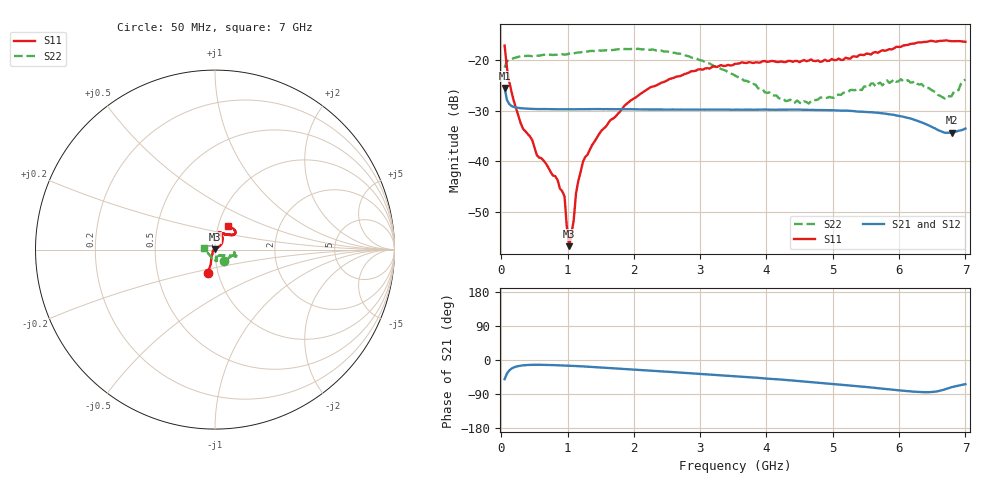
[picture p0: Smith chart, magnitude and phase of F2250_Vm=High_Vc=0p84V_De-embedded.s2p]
! Integrated Device Technology
! Corporate Headquarters
! 6024 Silver Creek Valley Road
! San Jose, CA 95138  USA
! Phone:  1-408-284-8200
! Toll Free:  1-800-223-1366
! Webpage:  http://www.idt.com/
! Timing and RF Division
! 515 Groton Road, Suite 102
! Westford, MA 01886-6024
! Device:  F2250
! Description: Voltage Variable RF Attenuator
! Frequency:  50.0 -  6000.00 MHz
! Package:  3x3 mm Thin QFN Plastic Package: 16 pin
! Ports:  2 RF, 3 DC
!  Pin  1  = GND
!  Pin  2  = NC
!  Pin  3  = RF1  = Port 1
!  Pin  4  = NC
!  Pin  5  = GND
!  Pin  6  = GND
!  Pin  7  = GND
!  Pin  8  = GND
!  Pin  9  = NC
!  Pin 10  = RF2  = Port 2
!  Pin 11  = NC
!  Pin 12  = GND
!  Pin 13  = GND
!  Pin 14  = VCNTRL
!  Pin 15  = VDD
!  Pin 16  = VMODE
! Vcntrl:  0.840 Volts
! Vmode:  +3.300 Volts
! Vdd:  +3.30  Volts
! Current:  1.308 mA
! Data:  The device was measured on a the F2250 evaluation board which has
!  individual transmission lines to the RF pins.  Data was collected
!  using a calibrated network analyzer.  The evaluation board was
!  de-embedded using a TRL calibration technique.
!  The reference plane is the edge of the package pin.
! Misc:  SN 10
!  Action Tracker AT0258
! Date Measured:  2014-11-26
! Date:  2015-10-15  MJV
! Note:
!  Integrated Device Technology supplies this data as a sample of measured
!  data at the package pin for this product.  Your particular data for this
!  product may vary.
!  Data was taken at 25 degrees C.
!  Integrated Device Technology reserves the right to change this data at anytime.
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# GHz S dB R 50
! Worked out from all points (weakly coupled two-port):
!   201 points, 50 MHz to 7 GHz, reference 50 ohm
!   highest |S21| = -25.53 dB at 50 MHz (marker M1); lowest = -34.4 dB at 6.792 GHz (marker M2)
!   lowest |S11| = -56.7 dB at 1.023 GHz (marker M3), VSWR 1.00, Z = 49.9 + j0.128 ohm
!   |S11| at or under -10 dB: start of sweep to end of sweep
!   |S22| runs from -28.6 to -17.8 dB; largest |S21 - S12| = 0.00014
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0.05  -17.15 -107.5  -25.53 -50.6  -25.52 -50.6  -21.52 -51.9
0.1195  -24.23 -110.3  -28.70 -27.7  -28.71 -27.7  -19.98 -15.0
0.29325  -32.52 -123.7  -29.53 -14.9  -29.50 -14.9  -19.22 -9.3
0.5365  -38.78 -149.6  -29.68 -12.7  -29.68 -12.7  -19.16 -9.0
0.8145  -42.95 171.8  -29.73 -13.6  -29.72 -13.6  -19.00 -12.1
0.9535  -46.90 174.9  -29.74 -14.5  -29.76 -14.5  -18.96 -13.8
0.98825  -52.90 169.1  -29.75 -14.8  -29.74 -14.8  -18.88 -14.2
1.023  -56.74 117.8  -29.74 -15.1  -29.72 -15.1  -18.76 -14.2
1.0925  -51.61 52.9  -29.73 -15.6  -29.73 -15.6  -18.70 -14.7
1.12725  -46.27 41.7  -29.73 -15.9  -29.72 -15.9  -18.59 -15.2
1.2315  -40.09 32.1  -29.72 -16.9  -29.72 -16.9  -18.39 -16.6
1.5095  -33.96 36.1  -29.71 -19.9  -29.71 -19.9  -18.19 -17.4
1.857  -29.03 36.8  -29.72 -23.7  -29.71 -23.7  -17.84 -18.5
2.37825  -24.75 45.1  -29.77 -29.5  -29.77 -29.5  -18.08 -18.8
3.525  -20.76 70.9  -29.82 -43.0  -29.81 -43.0  -23.07 -29.1
4.2895  -20.43 75.2  -29.81 -52.7  -29.80 -52.8  -28.12 -56.3
4.7065  -20.18 71.5  -29.86 -58.7  -29.84 -58.7  -27.86 -74.5
5.85325  -17.86 40.1  -30.73 -77.4  -30.72 -77.6  -24.53 -81.0
6.2355  -16.75 38.6  -31.85 -83.7  -31.83 -83.8  -24.20 -89.4
6.68725  -16.16 47.5  -34.36 -77.8  -34.36 -77.9  -27.59 -142.7
6.7915  -16.31 50.9  -34.37 -71.7  -34.32 -72.0  -27.17 -162.0
7  -16.41 62.0  -33.54 -63.8  -33.52 -63.9  -23.87 171.5
